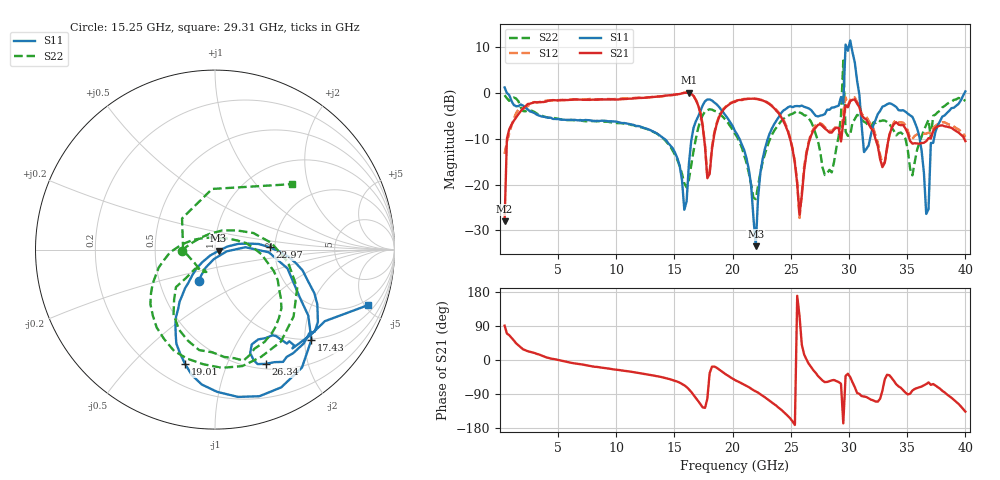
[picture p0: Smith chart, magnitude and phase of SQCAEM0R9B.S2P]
! Network Analyzer HP8722ES.07.66: Jul 25, 2000 Serial No. US39175408
! 26 Oct 2004  09:55:45
! Frequency  S11  S21  S12  S22
# HZ  S  DB R  50
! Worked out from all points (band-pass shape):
!   201 points, 400 MHz to 40 GHz, reference 50 ohm
!   highest |S21| = 0.12 dB at 16.24 GHz (marker M1); lowest = -28.0 dB at 400 MHz (marker M2)
!   |S21| within 3 dB of the highest: 2.184 GHz to 17.06 GHz (14.87 GHz wide, 155 % of centre); 19.49 GHz to 23.39 GHz (3.904 GHz wide, 18.2 % of centre)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
!   lowest |S11| = -33.5 dB at 21.98 GHz (marker M3), VSWR 1.04, Z = 52.1 - j0.685 ohm
!   |S11| at or under -10 dB: 14.13 GHz to 16.47 GHz (2.339 GHz wide, 15.3 % of centre); 20.58 GHz to 23.02 GHz (2.435 GHz wide, 11.2 % of centre); 36.07 GHz to 37.3 GHz (1.226 GHz wide, 3.34 % of centre)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
!   |S22| runs from -23.2 to 7.1 dB; largest |S21 - S12| = 0.24
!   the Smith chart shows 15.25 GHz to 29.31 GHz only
!   S11 on the Smith chart (normalised r, x): 15.25 GHz: 0.79, -0.28; 17.43 GHz: 0.98, -2.15; 19.01 GHz: 0.32, -0.72; 22.97 GHz: 1.87, +0.05; 26.34 GHz: 0.56, -1.39; 29.31 GHz: 1.52, -5.23
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4e8  1.25 2.0  -28.05 90.7  -13.30 83.2  -0.45 -5.5
1.192e9  -2.60 -37.3  -6.05 51.7  -5.63 46.2  -0.95 -42.7
7.132e9  -5.97 -97.5  -1.46 -12.1  -1.42 -11.8  -6.08 -106.8
1.3666e10  -9.12 -114.5  -0.73 -43.5  -0.74 -42.0  -9.22 -150.1
1.525e10  -14.24 -117.5  -0.26 -57.1  -0.24 -55.0  -14.61 -177.7
1.624e10  -15.39 4.4  0.12 -77.4  0.12 -74.3  -18.91 70.0
1.7428e10  -2.67 -43.1  -7.34 -125.2  -6.95 -121.3  -4.81 -40.4
1.9012e10  -3.61 -104.6  -4.36 -29.0  -4.19 -27.0  -4.83 -119.7
2.02e10  -8.29 -122.0  -1.92 -53.0  -1.73 -50.3  -8.88 -156.6
2.1982e10  -33.47 -18.1  -1.23 -82.9  -1.28 -79.2  -23.18 67.6
2.2972e10  -10.33 2.5  -2.09 -102.9  -1.98 -98.2  -11.68 -5.8
2.6338e10  -3.14 -66.0  -13.30 1.8  -12.94 3.2  -4.93 -98.9
2.6932e10  -4.31 -71.2  -8.18 -26.9  -7.87 -25.4  -7.38 -122.7
2.9308e10  -0.86 -20.0  -10.57 -62.7  -10.29 -59.6  -4.96 40.2
2.9506e10  -2.29 4.9  -6.37 -167.2  -4.16 -150.1  7.13 32.4
2.9704e10  10.62 -16.5  -2.65 -42.0  -0.95 -29.0  -8.44 -62.8
3.01e10  11.53 -85.5  -1.80 -45.1  -1.47 -39.7  -9.20 -2.2
3.0496e10  6.71 -116.6  -1.43 -71.7  -0.94 -65.4  -5.68 -38.0
3.0694e10  2.68 37.4  -2.29 -87.1  -1.97 -81.7  -4.75 128.7
3.3466e10  -2.21 -55.5  -9.14 -40.2  -9.22 -34.8  -6.67 -152.3
3.6634e10  -26.43 158.5  -10.52 -63.5  -8.86 -65.3  -6.93 66.2
4e10  0.38 -20.2  -10.49 -136.2  -9.54 -130.4  -1.70 -5.8
